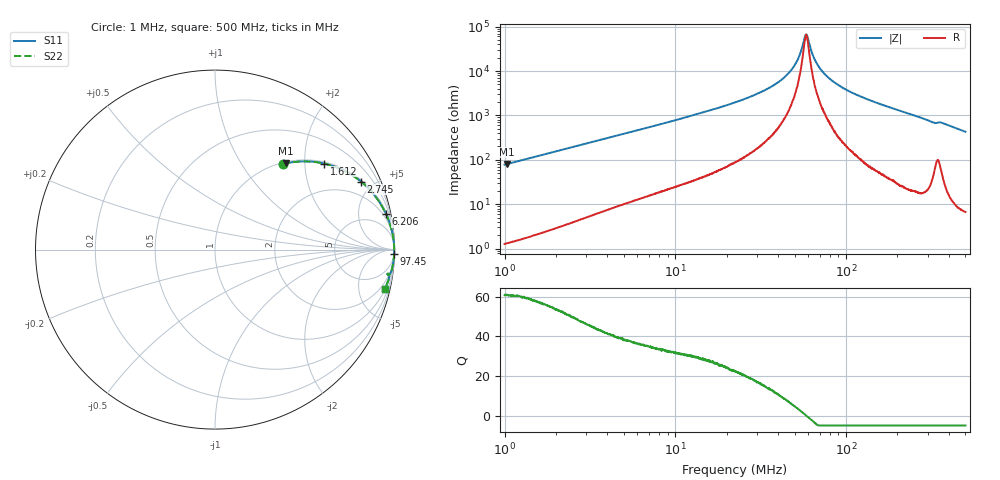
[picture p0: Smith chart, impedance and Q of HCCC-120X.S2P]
!s-Parameter Generated by FASTRON Sdn. Bhd.
!FASTRON P/N : HCCC-120X
!Keysight Technologies,E4991B,MY54100416,A.01.15
!Date: Mon Apr 06 15:29:44 2026
!Version  : Rev00 Mon Apr 06 15:29:44 2026
!Data & Calibration Information:
!PortZ  Port1:50+j0  Port2:50+j0
!When reading, reference impedance value at option line is always used.
! Remarks : This data is being provided solely for informational purposes.
!Freq	S11	S21	S12	S22
# Hz S dB R 50
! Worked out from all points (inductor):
!   1601 points, 1 MHz to 500 MHz, reference 50 ohm
!   read as one part in series: L = 12.4 uH near 1.032 MHz
!   highest Q = 60.9 at 1.036 MHz (marker M1), where L = 12.4 uH
!   self-resonance near 58.36 MHz
!   S11 on the Smith chart (normalised r, x): 1 MHz: 1.03, +1.56; 1.612 MHz: 1.04, +2.51; 2.745 MHz: 1.09, +4.25; 6.206 MHz: 1.27, +9.59; 97.45 MHz: 6, -80; 500 MHz: 1.13, -8.60
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1000000  -4.30 51.5  -2.13 -37.6  -2.13 -37.6  -4.30 51.5
1035575  -4.11 50.5  -2.25 -38.5  -2.25 -38.5  -4.11 50.5
1612439  -2.21 38.2  -4.18 -50.8  -4.18 -50.8  -2.21 38.2
2745255  -0.94 25.0  -7.49 -63.8  -7.49 -63.8  -0.94 25.0
2820919  -0.89 24.4  -7.69 -64.4  -7.69 -64.4  -0.89 24.4
6206152  -0.23 11.7  -13.86 -76.7  -13.86 -76.7  -0.23 11.7
7957584  -0.15 9.2  -15.96 -79.1  -15.96 -79.1  -0.15 9.2
2.236068e7  -0.03 2.9  -25.89 -84.5  -25.89 -84.5  -0.03 2.9
3.388275e7  -0.02 1.5  -31.61 -84.6  -31.61 -84.6  -0.02 1.5
4.378357e7  -0.01 0.8  -37.35 -82.4  -37.35 -82.4  -0.01 0.8
5.094464e7  -0.01 0.4  -43.65 -75.9  -43.65 -75.9  -0.01 0.4
5.337536e7  -0.01 0.2  -46.97 -70.1  -46.97 -70.1  -0.01 0.2
5.679767e7  -0.01 0.1  -54.14 -40.6  -54.14 -40.6  -0.01 0.1
5.813687e7  -0.01 0.0  -56.38 -7.7  -56.38 -7.7  -0.01 0.0
5.973923e7  -0.01 -0.1  -54.96 34.2  -54.96 34.2  -0.01 -0.1
6.307767e7  -0.01 -0.2  -48.27 67.6  -48.27 67.6  -0.01 -0.2
6.738328e7  -0.01 -0.4  -43.44 77.2  -43.44 77.2  -0.01 -0.4
7.339442e7  -0.01 -0.6  -39.43 81.5  -39.43 81.5  -0.01 -0.6
8.278574e7  -0.01 -0.9  -35.69 83.8  -35.69 83.8  -0.01 -0.9
9.745486e7  -0.01 -1.4  -32.12 85.3  -32.12 85.3  -0.01 -1.4
1.77937e8  -0.03 -3.7  -23.82 84.9  -23.82 84.9  -0.03 -3.7
5e8  -0.26 -13.0  -12.93 76.1  -12.93 76.1  -0.26 -13.0
